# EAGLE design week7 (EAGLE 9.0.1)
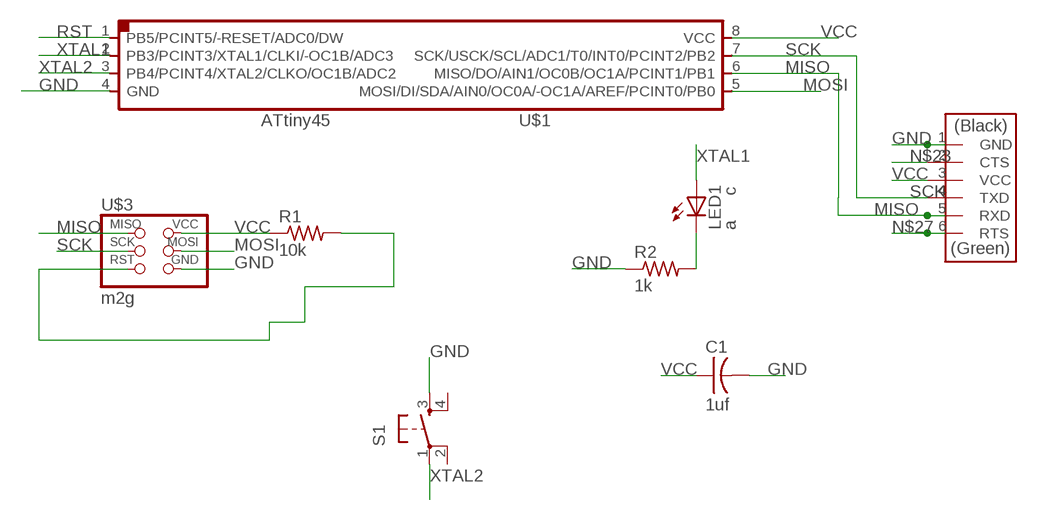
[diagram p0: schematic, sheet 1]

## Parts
C1  1uf  CAP-US1206FAB  [C1206FAB]
LED1  a c  LEDFAB1206  [LED1206FAB]
R1  10k  RES-US1206FAB  [R1206FAB]
R2  1k  RES-US1206FAB  [R1206FAB]
S1  6MM_SWITCH6MM_SWITCH  [6MM_SWITCH]
U$1  tt45  ATTINY45SI  [SOIC8]
U$3  m2g  AVRISPSMD  [2X03SMD]
U$4  FTDI-SMD-HEADER  [1X06SMD]

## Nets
GND: C1.2 R2.1 S1.3(S) U$1.4(GND) U$3.6(GND) U$4.1(GND)
MISO: U$1.6(MISO/DO/AIN1/OC0B/OC1A/PCINT1/PB1) U$3.1(MISO) U$4.5(RXD)
MOSI: U$1.5(MOSI/DI/SDA/AIN0/OC0A/-OC1A/AREF/PCINT0/PB0) U$3.4(MOSI)
N$1: LED1.2(C) R2.2
N$23: U$4.2(CTS)
N$27: U$4.6(RTS)
RST: R1.2 U$1.1(PB5/PCINT5/-RESET/ADC0/DW) U$3.5(RST)
SCK: U$1.7(SCK/USCK/SCL/ADC1/T0/INT0/PCINT2/PB2) U$3.3(SCK) U$4.4(TXD)
VCC: C1.1 R1.1 U$1.8(VCC) U$3.2(VCC) U$4.3(VCC)
XTAL1: LED1.1(A) U$1.2(PB3/PCINT3/XTAL1/CLKI/-OC1B/ADC3)
XTAL2: S1.1(P) U$1.3(PB4/PCINT4/XTAL2/CLKO/OC1B/ADC2)
Unconnected: S1.2(P1) S1.4(S1)

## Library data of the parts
C1 = fab:CAP-US
LED1 = fab:LED: LED
R1 R2 = fab:RES-US: Resistor (US Symbol)
S1 = fab:6MM_SWITCH: OMRON SWITCH
U$1 = fab:ATTINY45
U$3 = fab:AVRISP
U$4 = fab:FTDI-SMD-HEADER

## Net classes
0 default: width 0.4 mm, drill 0.4 mm, clearance 0.4 mm

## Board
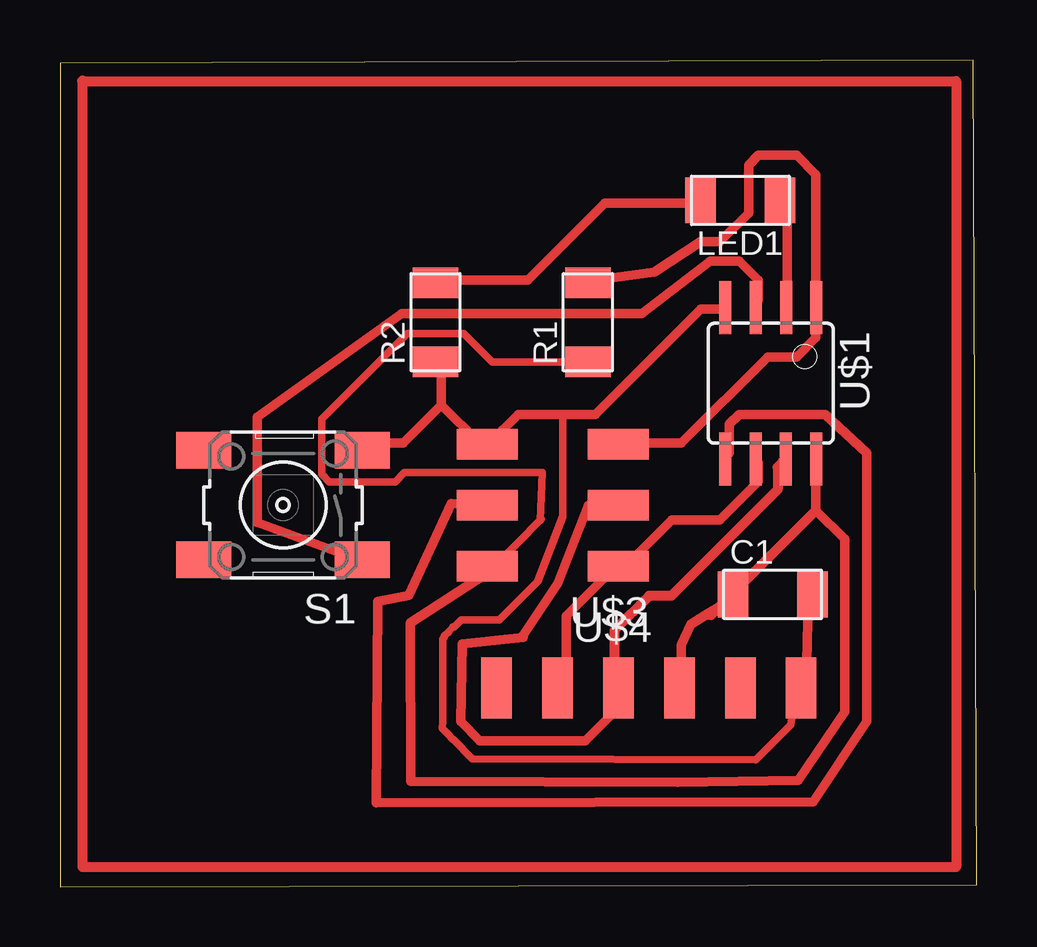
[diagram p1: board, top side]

Size 38.19 x 34.46 mm. Coordinates in mm from the lower left corner, seen from the top.
Outline: 0.02,0 38.19,0.08 38.05,34.46 0,34.32 0.02,0
Copper layers (1*16): Top 0.035mm / dielectric 1.5mm / Bottom 0.035mm
Design rules "default": minimum track width 6mil, minimum drill 0.35mm, track to track 6mil, track to pad 6mil, pad to pad 6mil, via to via 6mil, smd to smd 6mil, copper to edge 40mil, drill to drill 6mil, minimum pad ring 10mil, minimum via ring 8mil, stop-mask expansion 4mil, vias tented up to drill 0mil, thermal gap 10mil

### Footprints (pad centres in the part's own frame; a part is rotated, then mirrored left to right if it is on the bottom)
C1206FAB = smd 1.27 x 1.905: 1 -1.651,0; 2 1.651,0
LED1206FAB = smd 1.27 x 1.905: 1 -1.651,0; 2 1.651,0
R1206FAB = smd 1.27 x 1.905: 1 -1.651,0; 2 1.651,0
6MM_SWITCH = smd 2.286 x 1.524: 1 -3.302,2.286; 2 3.302,2.286; 3 -3.302,-2.286; 4 3.302,-2.286
SOIC8 = smd 0.5 x 2.2: 1 -1.905,-3.154; 2 -0.645,-3.154; 3 0.625,-3.154; 4 1.895,-3.154; 5 1.905,3.154; 6 0.635,3.154; 7 -0.635,3.154; 8 -1.905,3.154
2X03SMD = smd 2.54 x 1.27: 1 -2.54,2.54; 2 2.92,2.54; 3 -2.54,0; 4 2.92,0; 5 -2.54,-2.54; 6 2.92,-2.54
1X06SMD = smd 2.54 x 1.27: 1 0,6.35; 2 0,3.81; 3 0,1.27; 4 0,-1.27; 5 0,-3.81; 6 0,-6.35

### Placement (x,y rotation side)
C1  29.69,12.18 0 top
LED1  28.34,28.6 180 top
R1  21.99,23.52 90 top
R2  15.64,23.52 90 top
S1  9.29,15.9 180 top
U$1  29.61,20.98 180 top
U$3  20.72,15.9 180 top
U$4  24.53,8.28 270 top

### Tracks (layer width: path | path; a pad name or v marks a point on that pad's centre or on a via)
GND
  Top 0.305: U$4.1 30.48,7.01 30.44,6.75 28.99,5.29 17.18,5.33 16.38,6.14 16.37,6.14 16.16,6.36 15.94,6.57 15.94,6.58 15.94,6.59 15.94,6.89 15.94,10.31 16.01,10.39 16.01,10.44 16.21,10.62 16.37,10.83 16.43,10.83 16.71,11.12 18.3,11.12 19.91,12.73 20.95,15.43 20.95,19.68
  Top 0.4: 15.89,20.08 15.89,21.68 R2.1 | 15.89,20.08 17.49,18.48 U$3.6 17.89,18.48 19.09,19.68 20.95,19.68 22.29,19.68 26.69,24.08 27.49,24.08 U$1.4 | 15.89,20.08 14.29,18.48 12.69,18.48 S1.3 | C1.2 31.17,11.9 31.09,8.48 U$4.1
MISO
  Top 0.4: U$1.6 29.09,17.68 29.09,16.88 27.49,15.28 25.49,15.28 23.49,13.28 U$3.1 23.09,13.28 21.09,11.28 21.09,8.48 U$4.5
MOSI
  Top 0.4: U$1.5 27.89,18.08 27.89,19.28 28.29,19.68 31.89,19.68 33.61,18.08 33.61,6.88 31.38,3.53 13.17,3.49 13.23,11.89 14.52,12.14 16.3,15.97 U$3.4
N$1
  Top 0.4: R2.2 15.89,25.28 19.49,25.28 22.69,28.48 26.29,28.48 LED1.2
N$2
  Top 0.406: 0.92,33.58 37.34,33.58 37.34,0.81 0.95,0.81 0.95,33.61
RST
  Top 0.4: R1.2 22.29,25.28 24.76,25.62 26.69,26.88 27.49,26.88 28.69,28.08 28.69,30.08 29.09,30.48 30.69,30.48 31.49,29.68 31.49,24.48 U$1.1 31.49,24.08 31.49,22.88 30.69,22.08 29.49,22.08 25.89,18.48 23.49,18.48 U$3.5
SCK
  Top 0.4: 23.49,7.68 23.09,8.08 U$4.4 23.49,7.68 | 23.49,7.68 21.89,6.08 17.49,6.08 16.69,6.88 16.76,10.11 19.31,10.39 19.28,10.45 20.75,12.63 22,15.88 22.55,16.15 22.71,15.74 23.09,15.68 U$3.3
  Top 0.406: 23.09,8.08 23.09,10.68 24.55,12.13 25.48,12.13 29.9,16.55 29.9,17.48 U$1.7
VCC
  Top 0.305: 17.49,13.28 18.05,13.29 20.05,15.32 20,15.26 20.09,17.26 19.14,17.26 14.35,17.26 13.97,16.88 11.22,16.88 10.9,17.2 10.9,19.5 14.46,23.06 16.83,23.06 18.01,21.87 R1.1
  Top 0.4: C1.1 28.13,12.06 26.91,11.32 26.27,10.94 25.89,10.08 25.89,8.48 U$4.3 | U$1.8 31.49,17.68 31.49,15.68 32.69,14.48 32.69,7.28 30.76,4.42 25.75,4.34 14.61,4.38 14.6,11 18.09,13.27 17.49,13.28 U$3.2
  Top 0.406: 31.49,15.68 27.13,11.32 26.91,11.32
XTAL1
  Top 0.4: LED1.1 30.29,28.48 30.29,24.48 U$1.2
XTAL2
  Top 0.4: U$1.3 29.09,24.48 29.09,25.28 28.29,26.08 27.09,26.08 24.24,23.89 14.24,23.89 8.22,19.57 8.22,15.17 12.29,13.68 S1.1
